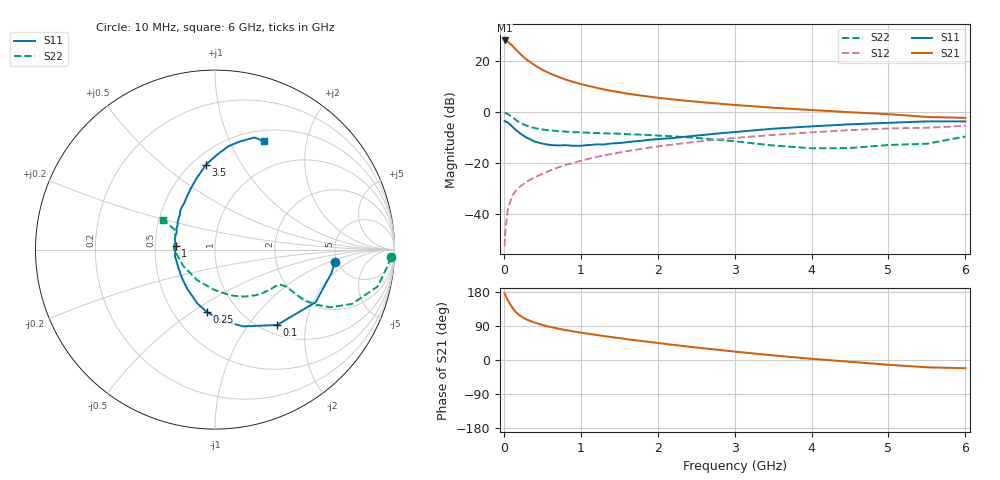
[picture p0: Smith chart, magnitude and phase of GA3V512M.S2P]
! Infineon Technologies  Discrete & RF Semiconductors
! BF775
! Si NPN RF Bipolar Junction Transistor in SOT23
! VCE = 3.5 V  IC = 12 mA
! Common Emitter S-Parameters:  May  1996
# GHz  S  MA  R  50
!  f  S11  S21  S12  S22
! GHz  MAG  ANG  MAG  ANG  MAG  ANG  MAG  ANG
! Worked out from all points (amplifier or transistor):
!   36 points, 10 MHz to 6 GHz, reference 50 ohm
!   highest |S21| = 28.1 dB at 10 MHz (marker M1)
!   |S21| within 3 dB of that: start of sweep to 139.3 MHz
!   unconditionally stable (mu >= 1): 496.6 MHz to 3.175 GHz
!   at 250 MHz: K = 0.74, MSG = 25.0 dB, |S12| = -28.2 dB
!   at 1.4 GHz: K = 1.11, MAG = 10.3 dB, |S12| = -16.3 dB
!   at 6 GHz: K = 0.95, MSG = 1.6 dB, |S12| = -5.3 dB
!   S11 on the Smith chart (normalised r, x): 10 MHz: 4.77, -1.15; 100 MHz: 1.16, -1.39; 250 MHz: 0.72, -0.58; 1 GHz: 0.64, +0.03; 3.5 GHz: 0.58, +0.71; 6 GHz: 0.63, +1.35
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0.01  0.6701 -5.7  25.35 175.4  0.0024 88.7  0.9804 -2.5
0.02  0.6625 -11.3  25.22 170.7  0.005 84.1  0.9672 -5.2
0.05  0.6329 -27.6  24.16 158.3  0.0122 77.5  0.9301 -12.7
0.1  0.5438 -50.6  20.72 141.2  0.0217 70.4  0.8215 -21.6
0.15  0.4561 -69.7  17.25 127.6  0.0288 65.1  0.7201 -26.5
0.2  0.3991 -84.5  14.51 118.7  0.034 63.5  0.6411 -28.6
0.25  0.3516 -97.0  12.27 111.7  0.0389 62.6  0.5841 -29.3
0.3  0.3161 -108.0  10.64 106.4  0.0443 63.2  0.5435 -29.2
0.4  0.2675 -125.4  8.325 98.8  0.0531 64.3  0.4899 -28.4
0.5  0.2433 -138.8  6.763 92.4  0.0622 65.6  0.4586 -27.6
0.6  0.2294 -151.6  5.74 87.5  0.0723 66.0  0.4411 -27.5
0.7  0.2238 -162.1  4.978 83.0  0.0824 66.3  0.4278 -27.8
0.8  0.2265 -170.7  4.377 79.2  0.0924 66.0  0.4175 -28.0
1  0.221 174.2  3.565 72.3  0.1122 65.8  0.4041 -29.3
1.1  0.2282 167.2  3.275 69.2  0.1226 65.3  0.3976 -30.7
1.3  0.2339 155.8  2.796 63.3  0.1432 63.8  0.3879 -32.9
1.6  0.2594 143.1  2.321 54.9  0.1734 61.4  0.3731 -37.5
2.2  0.3127 122.9  1.776 40.0  0.234 55.4  0.338 -49.0
3.5  0.4763 96.0  1.227 12.2  0.3597 39.5  0.2237 -91.6
4.5  0.5807 82.6  1.001 -4.7  0.4464 26.3  0.1992 -152.7
5.5  0.6619 70.6  0.809 -19.3  0.4973 11.5  0.2421 154.3
6  0.6619 65.5  0.775 -21.7  0.5417 7.4  0.3348 150.0
